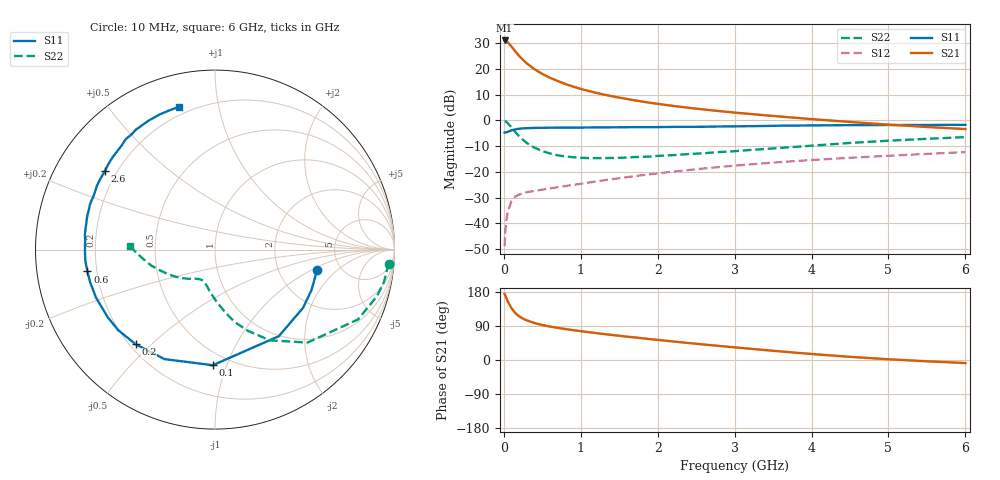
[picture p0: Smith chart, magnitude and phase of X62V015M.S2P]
! SIEMENS Small Signal Semiconductors
! BFP193W
! Si NPN RF Bipolar Junction Transistor in SOT343
! VCE = 2 V  IC = 15 mA
! Common Emitter S-Parameters:  April 1994
# GHz  S  MA  R  50
!  f  S11  S21  S12  S22
! GHz  MAG  ANG  MAG  ANG  MAG  ANG  MAG  ANG
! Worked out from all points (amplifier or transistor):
!   40 points, 10 MHz to 6 GHz, reference 50 ohm
!   highest |S21| = 31.1 dB at 10 MHz (marker M1)
!   |S21| within 3 dB of that: start of sweep to 116.1 MHz
!   unconditionally stable (mu >= 1): 1.03 GHz to 4.076 GHz
!   at 200 MHz: K = 0.30, MSG = 26.9 dB, |S12| = -28.8 dB
!   at 1.5 GHz: K = 1.11, MAG = 13.6 dB, |S12| = -22.5 dB
!   at 6 GHz: K = 0.93, MSG = 4.5 dB, |S12| = -12.3 dB
!   S11 on the Smith chart (normalised r, x): 10 MHz: 3.34, -1.14; 100 MHz: 0.41, -0.89; 200 MHz: 0.22, -0.45; 600 MHz: 0.16, -0.08; 2.6 GHz: 0.15, +0.31; 6 GHz: 0.16, +0.77
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0.01  0.5801 -11.3  35.8 174.0  0.0036 84.7  0.9699 -4.6
0.02  0.583 -22.9  35.58 169.5  0.0073 80.7  0.9588 -10.9
0.03  0.5882 -33.5  35.03 164.6  0.0107 78.0  0.9385 -16.1
0.05  0.5993 -53.6  33.08 155.0  0.0168 69.5  0.8871 -26.0
0.1  0.6443 -91.1  27.18 136.5  0.0273 53.4  0.7309 -45.1
0.15  0.672 -114.8  21.87 123.6  0.0332 44.7  0.5922 -58.7
0.2  0.6881 -129.9  17.83 115.1  0.0362 39.8  0.4898 -67.8
0.25  0.7017 -140.3  14.99 109.0  0.0387 37.0  0.4186 -74.7
0.3  0.7065 -147.8  12.76 104.4  0.0403 35.4  0.3624 -79.9
0.4  0.715 -158.1  9.855 97.5  0.0428 34.9  0.2948 -87.8
0.5  0.7188 -165.2  8.01 92.3  0.0452 36.2  0.254 -93.6
0.6  0.7212 -170.3  6.723 88.2  0.0476 37.6  0.2276 -98.5
0.8  0.7245 -178.2  5.097 81.6  0.0532 40.6  0.1994 -105.1
1.1  0.7295 173.5  3.748 73.5  0.062 44.8  0.1851 -112.6
1.3  0.7314 168.7  3.179 68.5  0.0685 46.9  0.1856 -116.2
1.6  0.7371 162.3  2.607 61.6  0.0789 48.9  0.19 -120.7
2.2  0.7482 151.4  1.917 48.9  0.101 50.4  0.2116 -130.0
2.6  0.753 144.6  1.633 40.9  0.1165 50.0  0.2304 -136.0
3.2  0.7726 134.9  1.335 29.8  0.1395 47.8  0.2661 -145.3
4.5  0.8083 117.2  0.934 8.3  0.1879 40.8  0.3652 -165.8
5.5  0.8161 108.3  0.745 -3.4  0.2236 35.0  0.4396 -177.8
6  0.8212 104.1  0.68 -8.0  0.2423 32.4  0.4737 177.5
